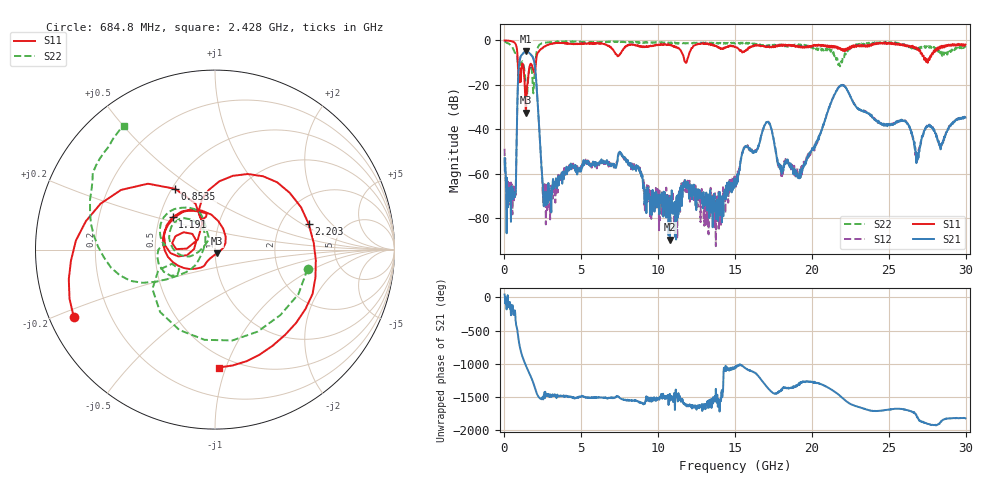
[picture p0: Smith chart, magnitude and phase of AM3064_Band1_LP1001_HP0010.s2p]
# Hz S DB R 50.0
!freq dBS11 angS11 dBS21 angS21 dBS12 angS12 dBS22 angS22
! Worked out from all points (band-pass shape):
!   1600 points, 10 MHz to 29.98 GHz, reference 50 ohm
!   highest |S21| = -4.90 dB at 1.397 GHz (marker M1); lowest = -89.7 dB at 10.77 GHz (marker M2)
!   |S21| within 3 dB of the highest: 1.027 GHz to 1.863 GHz (836.3 MHz wide, 57.9 % of centre)
!   lowest |S11| = -32.6 dB at 1.397 GHz (marker M3), VSWR 1.05, Z = 51 - j2.16 ohm
!   |S11| at or under -10 dB: 865.8 MHz to 2.046 GHz (1.18 GHz wide, 81.1 % of centre); 11.78953 GHz to 11.83828 GHz (48.75 MHz wide, 0.413 % of centre); 27.52354 GHz to 27.53577 GHz (12.22 MHz wide, 0.0444 % of centre)
!   |S22| runs from -24.4 to -0.3 dB; largest |S21 - S12| = 0.0079
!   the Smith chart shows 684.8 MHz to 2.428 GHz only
!   S11 on the Smith chart (normalised r, x): 684.8 MHz: 0.07, -0.22; 853.5 MHz: 0.52, +0.42; 1.191 GHz: 0.58, +0.23; 2.203 GHz: 2.83, +1.15; 2.428 GHz: 0.41, -0.95
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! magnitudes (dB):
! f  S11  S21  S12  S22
! 10 MHz  -0.1  -53.0  -48.8  -0.3
! 272.4 MHz  -0.2  -66.6  -64.1  -1.5
! 684.8 MHz  -1.2  -70.6  -69.0  -5.6
! 853.5 MHz  -7.9  -24.8  -24.8  -9.5
! 1.191 GHz  -10.5  -6.1  -6.0  -9.5
! 1.397 GHz  -32.6  -4.9  -4.9  -21.0
! 1.903 GHz  -13.8  -8.7  -8.7  -21.4
! 2.203 GHz  -5.3  -32.8  -32.7  -2.7
! 2.428 GHz  -3.6  -58.9  -58.2  -1.4
! 2.822 GHz  -2.0  -67.6  -64.0  -0.8
! 5.015 GHz  -1.4  -57.0  -57.6  -0.6
! 7.564 GHz  -5.8  -50.7  -50.8  -0.6
! 10 GHz  -2.0  -70.5  -68.7  -0.9
! 10.77 GHz  -2.0  -89.7  -72.3  -1.1
! 15 GHz  -2.9  -64.1  -64.3  -1.4
! 17.07 GHz  -2.8  -36.9  -36.7  -2.3
! 17.99 GHz  -2.4  -59.0  -61.0  -2.3
! 19.99 GHz  -2.8  -49.3  -49.9  -3.0
! 21.88 GHz  -4.0  -20.4  -20.4  -9.7
! 25 GHz  -1.0  -37.8  -38.1  -1.1
! 26.85 GHz  -4.3  -54.0  -52.8  -3.1
! 29.98 GHz  -1.9  -34.8  -35.0  -3.2
